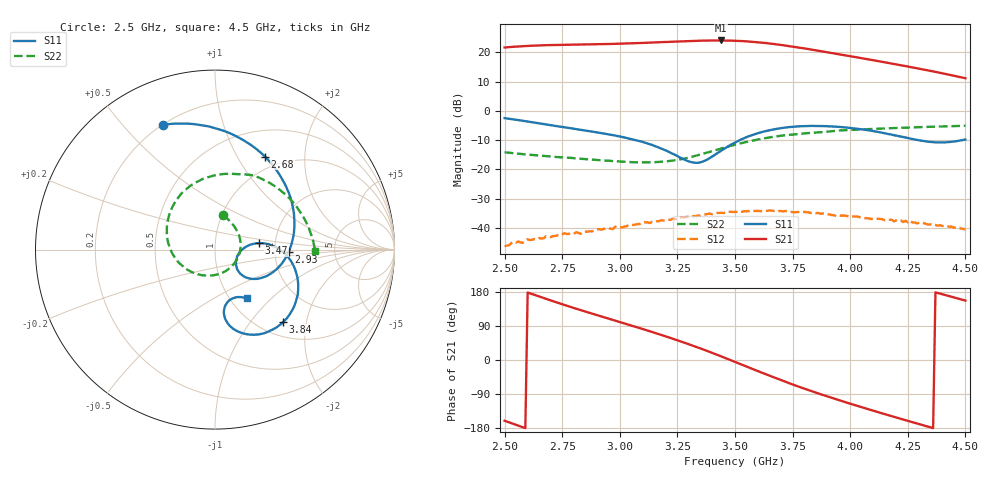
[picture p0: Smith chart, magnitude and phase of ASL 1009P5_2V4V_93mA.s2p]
!ASL 1009P5 : Low Noise Amplifier S-parameter data 2.5-4.5 GHz
!Bias conditions Vd1=2V, Vd2=4V, Total current=93 mA
!Date: Tuesday, January 09, 2007 14:23:47
!S2P File: Measurements: S11, S21, S12, S22:
# Hz S  dB  R 50
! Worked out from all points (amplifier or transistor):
!   201 points, 2.5 GHz to 4.5 GHz, reference 50 ohm
!   highest |S21| = 24.1 dB at 3.44 GHz (marker M1)
!   |S21| within 3 dB of that: start of sweep to 3.823 GHz
!   unconditionally stable (mu >= 1): start of sweep to end of sweep
!   at 2.83 GHz: K = 3.62, MAG = 23.9 dB, |S12| = -42.1 dB
!   at 3.5 GHz: K = 1.60, MAG = 24.7 dB, |S12| = -34.5 dB
!   at 4.5 GHz: K = 8.92, MAG = 13.3 dB, |S12| = -40.5 dB
!   S11 on the Smith chart (normalised r, x): 2.5 GHz: 0.20, +0.65; 2.68 GHz: 0.83, +1.31; 2.93 GHz: 2.39, -0.07; 3.47 GHz: 1.64, +0.13; 3.84 GHz: 1.27, -1.47; 4.5 GHz: 1.19, -0.72
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2.5e9  -2.47 112.5  21.70 -160.3  -46.27 121.5  -14.16 76.8
2.59e9  -3.51 87.2  22.20 -179.8  -44.41 101.8  -14.86 64.2
2.68e9  -4.60 61.7  22.49 161.2  -42.85 85.0  -15.46 50.9
2.84e9  -6.57 19.3  22.72 129.8  -41.47 56.3  -16.40 22.9
2.93e9  -7.72 -1.6  22.86 113.0  -40.30 40.6  -16.94 3.5
3.05e9  -9.61 -25.3  23.12 90.9  -38.99 22.2  -17.53 -27.5
3.17e9  -12.55 -41.6  23.49 68.2  -37.70 -0.4  -17.49 -67.4
3.23e9  -14.67 -43.2  23.69 56.2  -36.82 -11.5  -17.00 -89.7
3.3e9  -17.29 -31.3  23.91 41.4  -36.21 -25.1  -15.93 -116.4
3.38e9  -16.62 -1.2  24.07 23.7  -35.29 -42.6  -14.24 -146.8
3.44e9  -13.61 8.3  24.11 9.6  -34.86 -56.8  -12.86 -168.4
3.47e9  -12.12 8.3  24.07 2.4  -34.50 -62.9  -12.21 -178.8
3.5e9  -10.80 6.5  24.01 -5.0  -34.54 -71.4  -11.56 171.3
3.58e9  -8.13 -3.8  23.62 -24.6  -34.21 -89.4  -10.10 146.3
3.67e9  -6.28 -18.8  22.88 -46.3  -34.25 -111.2  -8.80 121.4
3.76e9  -5.37 -34.1  21.88 -66.8  -34.64 -129.7  -7.96 99.7
3.84e9  -5.14 -46.8  20.88 -83.7  -34.88 -147.9  -7.44 83.2
3.92e9  -5.31 -58.1  19.82 -99.9  -35.64 -161.9  -6.93 68.8
4e9  -5.81 -67.7  18.73 -115.3  -36.23 -177.6  -6.51 56.1
4.17e9  -7.93 -81.1  16.35 -146.4  -37.23 152.1  -5.94 33.3
4.33e9  -10.43 -76.7  13.99 -174.7  -38.68 126.1  -5.48 15.4
4.5e9  -9.78 -57.1  11.18 156.8  -40.51 100.6  -5.08 -1.1
